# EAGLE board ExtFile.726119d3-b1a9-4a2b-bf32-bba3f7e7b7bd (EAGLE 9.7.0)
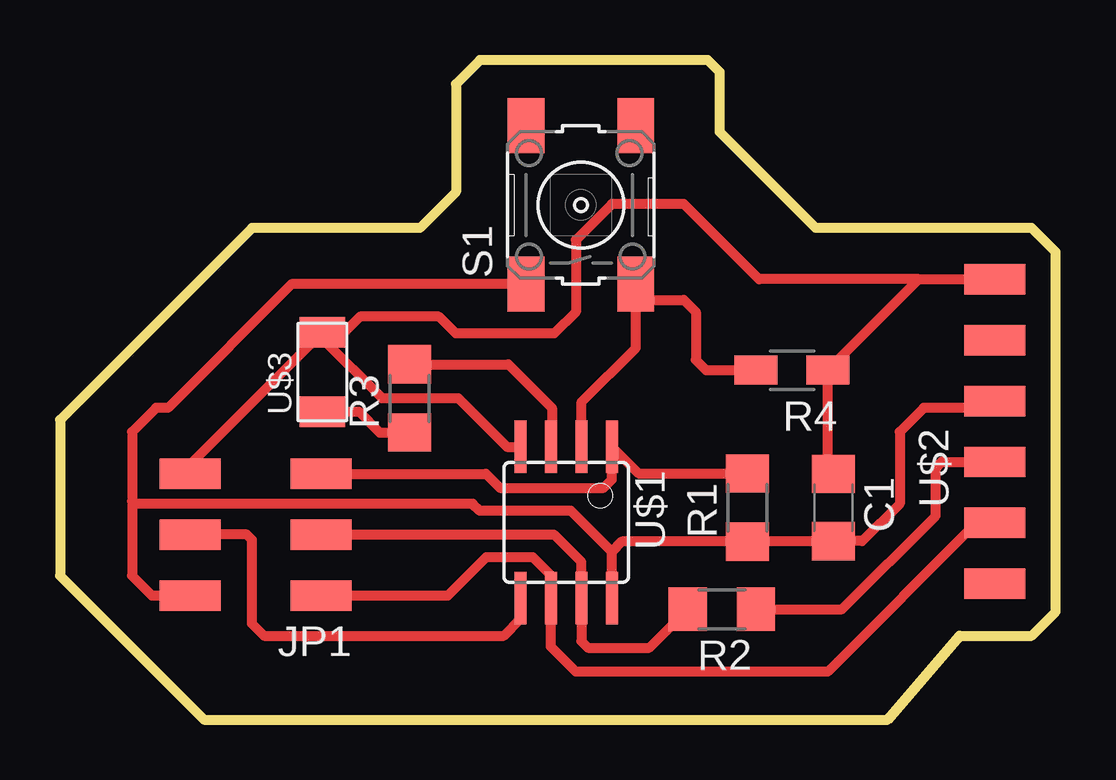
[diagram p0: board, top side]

Size 41.5 x 27.5 mm. Coordinates in mm from the lower left corner, seen from the top.
Outline: 8,20.5 0,12.5 0,6 6,0 34.5,0 37.5,3.5 40.5,3.5 41.5,4.5 41.5,19.5 40.5,20.5 31.5,20.5 27.5,24.5 27.5,27 27,27.5 17.5,27.5 16.5,26.5 16.5,22 15,20.5 8,20.5
Copper layers (1*16): Top 0.035mm / dielectric 1.5mm / Bottom 0.035mm
Design rules "hello board desrules": minimum track width 16mil, minimum drill 0.35mm, track to track 0.41mm, track to pad 0.41mm, pad to pad 0.41mm, via to via 0.41mm, smd to smd 6mil, copper to edge 0.41mm, drill to drill 0.41mm, minimum pad ring 10mil, minimum via ring 8mil, stop-mask expansion 4mil, vias tented up to drill 0mil, thermal gap 0.41mm

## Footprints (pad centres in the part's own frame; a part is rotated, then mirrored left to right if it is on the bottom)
C1206 = smd 1.6 x 1.8: 1 -1.4,0; 2 1.4,0
2X03SMD = smd 2.54 x 1.27: 1 -2.54,2.54; 2 2.92,2.54; 3 -2.54,0; 4 2.92,0; 5 -2.54,-2.54; 6 2.92,-2.54
R1206 = smd 1.6 x 1.803: 1 -1.422,0; 2 1.422,0
R1206W = smd 1.8 x 1.2: 1 -1.499,0; 2 1.499,0
6MM_SWITCH = smd 2.286 x 1.524: 1 -3.302,2.286; 2 3.302,2.286; 3 -3.302,-2.286; 4 3.302,-2.286
SOIC8 = smd 0.5 x 2.2: 1 -1.905,-3.154; 2 -0.645,-3.154; 3 0.625,-3.154; 4 1.895,-3.154; 5 1.905,3.154; 6 0.635,3.154; 7 -0.635,3.154; 8 -1.905,3.154
1X06SMD = smd 2.54 x 1.27: 1 0,6.35; 2 0,3.81; 3 0,1.27; 4 0,-1.27; 5 0,-3.81; 6 0,-6.35
LED1206FAB = smd 1.27 x 1.905: 1 -1.651,0; 2 1.651,0

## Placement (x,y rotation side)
C1  1uf  [C1206]  32.24,8.84 270 top
JP1  0  [2X03SMD]  8.34,7.71 180 top
R1  10k  [R1206]  28.66,8.84 90 top
R2  1k  [R1206]  27.59,4.6 180 top
R3  1k  [R1206]  14.57,13.39 90 top
R4  10k  [R1206W]  30.51,14.57 180 top
S1  0  [6MM_SWITCH]  21.71,21.45 90 top
U$1  UC_ATTINY45SI  [SOIC8]  21.1,8.22 180 top
U$2  CONN_06_FTDI-SMD-HEADER  [1X06SMD]  38.96,12.01 0 top
U$3  LEDFAB1206  [LED1206FAB]  10.93,14.49 90 top

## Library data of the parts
C1 JP1 R4 U$2 = fab
R1-R3 S1 U$3 = eagle_fab
U$1 = fab; SPICEPREFIX: X

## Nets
GND: C1.1 JP1.6 R4.1 U$1.4 U$2.1 U$3.2
MOSI: JP1.4 U$1.5
N$1: R3.1 U$3.1
PB1: JP1.1 U$1.6 U$2.5
PB2: JP1.3 R2.2 U$1.7
PB3: R4.2 S1.3 U$1.2
PB4: R3.2 U$1.3
RST: JP1.5 R1.2 U$1.1
TXD: R2.1 U$2.4
VCC: C1.2 JP1.2 R1.1 S1.1 U$1.8 U$2.3

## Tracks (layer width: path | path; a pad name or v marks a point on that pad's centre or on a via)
GND
  Top 0.406: U$3.2 10.82,16.25 | 35.8,18.36 U$2.1 | 35.8,18.36 R4.1 32.01,10.47 C1.1 | 35.8,18.36 29.14,18.36 26,21.5 23,21.5 21.5,20 21.5,17 20.6,16.1 16.5,16.1 15.8,16.8 12.5,16.8 11.8,16.1 11.8,15.9 11.18,15.9 U$3.2 | U$3.2 5.42,10.63 JP1.6 | U$3.2 11.19,16.4 | U$3.2 10.93,15.88 13.42,13.4 16.6,13.4 18.63,11.37 U$1.4
MOSI
  Top 0.406: JP1.4 7.79,7.71 8,7.5 8,4 8.5,3.5 18.5,3.5 19.2,4.2 U$1.5
N$1
  Top 0.406: U$3.1 12.46,12.84 13.33,11.97 R3.1 14.1,11.5
PB1
  Top 0.406: JP1.1 16.17,5.17 17.78,6.78 19.7,6.78 20.47,6.01 U$1.6 20.47,3.03 21.5,2 32,2 38.2,8.2 U$2.5
PB2
  Top 0.406: R2.2 24.57,3 22,3 21.74,3.26 U$1.7 21.74,6.56 20.59,7.71 JP1.3
PB3
  Top 0.406: U$1.2 21.75,13.25 24,15.5 S1.3 24.65,17.5 26,17.5 26.5,17 26.5,15 26.93,14.57 R4.2
PB4
  Top 0.406: U$1.3 20.5,11.4 20.5,13 18.69,14.81 R3.2
RST
  Top 0.406: R1.2 24.12,10.26 U$1.1 23.01,10.01 22.66,9.66 18.34,9.66 17.75,10.25 JP1.5 11.32,9.82 11.36,9.82
TXD
  Top 0.406: R2.1 32.6,4.6 36.5,8.5 36.5,10.5 36.74,10.74 U$2.4
VCC
  Top 0.406: U$2.3 38.68,13 36,13 35,12 35,9 33.44,7.44 C1.2 28.68,7.44 R1.1 23.42,7.42 23,7 | 3,9.1 3,12 4,13 4.5,13 9.65,18.15 S1.1 | 3,9.1 3,6 3.83,5.17 JP1.2 | 23,7 21.3,8.7 17.5,8.7 17.2,9 3.1,9 3,9.1 | U$1.8 23.01,6.99 23,7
